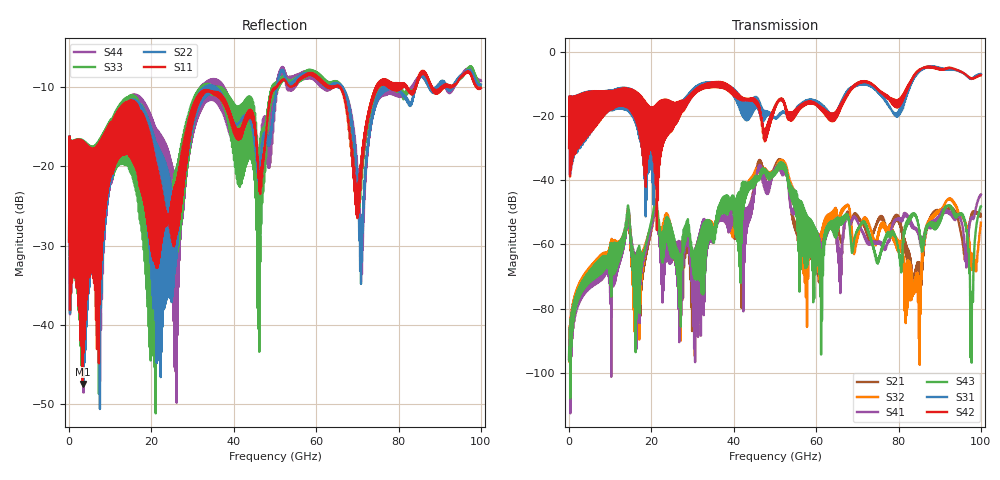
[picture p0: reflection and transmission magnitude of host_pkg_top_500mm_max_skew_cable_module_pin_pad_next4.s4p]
# Hz S RI R 50
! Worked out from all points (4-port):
!   10000 points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, 10 MHz to 100 GHz, reference 50 ohm
!   strongest paths, dB at 10 MHz, 25.01 GHz, 50.01 GHz, 75.01 GHz, 100 GHz:
!     S42: -29.9, -15.8, -16.8, -11.6, -7.2
!     S31: -29.9, -18.2, -20.6, -12.6, -6.9
!     S43: -95.7, -56.4, -36.9, -65.4, -48.1
!     S41: -95.7, -56.0, -36.2, -59.7, -44.4
!     S32: -95.8, -55.9, -36.7, -57.0, -53.2
!     S21: -95.7, -56.9, -35.4, -52.4, -51.2
!   lowest |S11| = -47.5 dB at 3.27 GHz (marker M1), VSWR 1.01, Z = 50.3 + j0.332 ohm
!   |S11| at or under -10 dB: start of sweep to 50.25 GHz; 65.92 GHz to 74.54 GHz (8.622 GHz wide, 12.3 % of centre); 88.1 GHz to 90.39 GHz (2.287 GHz wide, 2.56 % of centre)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
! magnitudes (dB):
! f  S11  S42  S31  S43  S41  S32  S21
! 10 MHz  -29.5  -29.9  -29.9  -95.7  -95.7  -95.8  -95.7
! 3.27 GHz  -47.5  -24.8  -22.4  -71.7  -73.2  -70.5  -71.9
! 51.61 GHz  -9.2  -14.7  -19.0  -35.0  -36.9  -33.6  -34.0
! 61.19 GHz  -9.3  -17.5  -16.2  -78.3  -62.6  -59.8  -67.3
! 92.1 GHz  -9.8  -5.0  -5.4  -47.8  -50.2  -45.8  -49.2
! 97.68 GHz  -8.6  -8.2  -8.4  -75.6  -51.7  -65.3  -50.7
! 100 GHz  -10.1  -7.2  -6.9  -48.1  -44.4  -53.2  -51.2
